(* Logix 5000 AddOnInstructionDefinition export EH_AL1323_8P_CommAOI; software revision 35.00 *)

TYPE EH_CommAOI_Data :
STRUCT
   Device_Comm_Error : BOOL;
   CommSuccess : BOOL;
   CommFailed : BOOL;
   CommTimeOut : BOOL;
   StateDone : BOOL;
   NewState : BOOL;
   OldState : SINT;
   PortSize : SINT;
   DevicePort : SINT;
   MaxState : SINT;
   State : SINT;
   VendorID : INT;
   DeviceID : DINT;
   CyclicData : INT[16];
   AcyclicData : DINT[8];
   ReplayIndex : INT;
   AOI_Diagnostic : DINT;
   ConnectionStatus : DINT;
   OutputData : INT[16];
END_STRUCT
END_TYPE

ADD_ON_INSTRUCTION EH_AL1323_8P_CommAOI   (* revision 1.0, vendor Endress+Hauser *)
// Ethenet/IP Comm AOI for 8 Port IFM AL 1323
// Revision note:
// First release of the IFM CommAOI with no array in the Tag Structure.
VAR_IN_OUT
   Master_InputTag : _0142:AL1323_43F9D57A:I:0; {required}
   Master_OutputTag : _0142:AL1323_F1871E46:O:0; {required}
   DataToSend : INT[10]; {required}
   CommAOIBusy : DINT; {required}
   ActiveComPort : DINT; {required}
   Send_Request : DINT; {required}
   CommError : INT; {required}
   DeviceData : EH_CommAOI_Data; {required}
END_VAR
VAR_INPUT
   iPortSize : INT; {required}
   iDevicePort : INT; {required}
   Master_Input_ConnectionFaulted : BOOL; {required}
END_VAR
VAR
   LocalChannel : DINT; {access None}
   LocalStep : DINT; {access None}
   cChannel : DINT; {access None}
   Port : SINT; {access None}
   count : SINT; {access None}
   PortSize : INT; {access None}
   ChannelData : DINT[15]; {access None}
   TONR_01 : FBD_TIMER; {access None}
   Calc_ConnectionStatus : INT; {access None}
   Calc_VID : INT; {access None}
   Calc_DID : INT; {access None}
   UsedState : INT; {access None}
   DataSendExecuted : BOOL; {access None}
   DataSize : SINT; {access None}
   RW_Input : SINT; {access None}
   RW_Step : SINT; {access None}
   TimerActive : BOOL; {access None}
   ExecuteCounter : DINT; {access None}
END_VAR

ROUTINE Logic   (* structured text *)
   //Create the Port Config 8P
   if iDevicePort > 0 and iDevicePort<9 then
   DeviceData.DevicePort := iDevicePort;
   else
   DeviceData.DevicePort := 0;
   end_if;
   
   DeviceData.PortSize := iPortSize;
   DeviceData.Device_Comm_Error := Master_Input_ConnectionFaulted;
   
   case DeviceData.PortSize of
   
   	0:
   		PortSize:= 1;
   	1:
   		PortSize:= 2;
   	2:
   		PortSize:= 4;
   	3:
   		PortSize:= 8;
   	4:
   		PortSize:= 16; //16 Int = 32Byte
   
   		DeviceData.AOI_Diagnostic.0 := 0;
   
   	else
   
   		DeviceData.AOI_Diagnostic.0 := 1;
   
   end_case;
   
   case DeviceData.DevicePort of
   
   	1:
   		//*********************************
   		//Device Connection Status within the Master
   		//*********************************
   
   		if Master_InputTag.Input_Data24 = 1
   		or Master_InputTag.Input_Data24 = 129 then
   
   			DeviceData.ConnectionStatus := 1; //Good
   
   		else
   
   			DeviceData.ConnectionStatus := 2; //Bad
   
   		end_if;
   
   		//*********************************
   		//Vendor ID
   		//*********************************
   
   		DeviceData.VendorID		:= Master_InputTag.Input_Data25;
   		DeviceData.VendorID.8	:= Master_InputTag.Input_Data25.8;
   		DeviceData.VendorID.9	:= Master_InputTag.Input_Data25.9;
   		DeviceData.VendorID.10	:= Master_InputTag.Input_Data25.10;
   		DeviceData.VendorID.11	:= Master_InputTag.Input_Data25.11;
   		DeviceData.VendorID.12	:= Master_InputTag.Input_Data25.12;
   		DeviceData.VendorID.13	:= Master_InputTag.Input_Data25.13;
   		DeviceData.VendorID.14	:= Master_InputTag.Input_Data25.14;
   		DeviceData.VendorID.15	:= Master_InputTag.Input_Data25.15;
   
   		//*********************************
   		//Device ID
   		//*********************************
   
   		DeviceData.DeviceID		:= Master_InputTag.Input_Data26;
   		DeviceData.DeviceID.8	:= Master_InputTag.Input_Data26.8;
   		DeviceData.DeviceID.9	:= Master_InputTag.Input_Data26.9;
   		DeviceData.DeviceID.10	:= Master_InputTag.Input_Data26.10;
   		DeviceData.DeviceID.11	:= Master_InputTag.Input_Data26.11;
   		DeviceData.DeviceID.12	:= Master_InputTag.Input_Data26.12;
   		DeviceData.DeviceID.13	:= Master_InputTag.Input_Data26.13;
   		DeviceData.DeviceID.14	:= Master_InputTag.Input_Data26.14;
   		DeviceData.DeviceID.15	:= Master_InputTag.Input_Data26.15;
   		DeviceData.DeviceID.16	:= Master_InputTag.Input_Data27.0;
   		DeviceData.DeviceID.17	:= Master_InputTag.Input_Data27.1;
   		DeviceData.DeviceID.18	:= Master_InputTag.Input_Data27.2;
   		DeviceData.DeviceID.19	:= Master_InputTag.Input_Data27.3;
   		DeviceData.DeviceID.20	:= Master_InputTag.Input_Data27.4;
   		DeviceData.DeviceID.21	:= Master_InputTag.Input_Data27.5;
   		DeviceData.DeviceID.22	:= Master_InputTag.Input_Data27.6;
   		DeviceData.DeviceID.23	:= Master_InputTag.Input_Data27.7;
   
   		//*********************************
   		//Cyclic Data Input
   		//*********************************
   
   		DeviceData.CyclicData[0] := Master_InputTag.Input_Data96;
   		DeviceData.CyclicData[1] := Master_InputTag.Input_Data97;
   		DeviceData.CyclicData[2] := Master_InputTag.Input_Data98;
   		DeviceData.CyclicData[3] := Master_InputTag.Input_Data99;
   		DeviceData.CyclicData[4] := Master_InputTag.Input_Data100;
   		DeviceData.CyclicData[5] := Master_InputTag.Input_Data101;
   		DeviceData.CyclicData[6] := Master_InputTag.Input_Data102;
   		DeviceData.CyclicData[7] := Master_InputTag.Input_Data103;
   		DeviceData.CyclicData[8] := Master_InputTag.Input_Data104;
   		DeviceData.CyclicData[9] := Master_InputTag.Input_Data105;
   		DeviceData.CyclicData[10] := Master_InputTag.Input_Data106;
   		DeviceData.CyclicData[11] := Master_InputTag.Input_Data107;
   		DeviceData.CyclicData[12] := Master_InputTag.Input_Data108;
   		DeviceData.CyclicData[13] := Master_InputTag.Input_Data109;
   		DeviceData.CyclicData[14] := Master_InputTag.Input_Data110;
   		DeviceData.CyclicData[15] := Master_InputTag.Input_Data111;
   
   
   		//*********************************
   		//Cyclic Data Output
   		//*********************************
   
   		Master_OutputTag.Output_Data24 := DeviceData.OutputData[0];
   		Master_OutputTag.Output_Data25 := DeviceData.OutputData[1];
   		Master_OutputTag.Output_Data26 := DeviceData.OutputData[2];
   		Master_OutputTag.Output_Data27 := DeviceData.OutputData[3];
   		Master_OutputTag.Output_Data28 := DeviceData.OutputData[4];
   		Master_OutputTag.Output_Data29 := DeviceData.OutputData[5];
   		Master_OutputTag.Output_Data30 := DeviceData.OutputData[6];
   		Master_OutputTag.Output_Data31 := DeviceData.OutputData[7];
   		Master_OutputTag.Output_Data32 := DeviceData.OutputData[8];
   		Master_OutputTag.Output_Data33 := DeviceData.OutputData[9];
   		Master_OutputTag.Output_Data34 := DeviceData.OutputData[10];
   		Master_OutputTag.Output_Data35 := DeviceData.OutputData[11];
   		Master_OutputTag.Output_Data36 := DeviceData.OutputData[12];
   		Master_OutputTag.Output_Data37 := DeviceData.OutputData[13];
   		Master_OutputTag.Output_Data38 := DeviceData.OutputData[14];
   		Master_OutputTag.Output_Data39 := DeviceData.OutputData[15];
   
   	2:
   		//*********************************
   		//Device Connection Status within the Master
   		//*********************************
   
   		if Master_InputTag.Input_Data33 = 1
   		or Master_InputTag.Input_Data33 = 129 then
   
   			DeviceData.ConnectionStatus := 1; //Good
   
   		else
   
   			DeviceData.ConnectionStatus := 2; //Bad
   
   		end_if;
   
   		//*********************************
   		//Vendor ID
   		//*********************************
   
   		DeviceData.VendorID		:= Master_InputTag.Input_Data34;
   		DeviceData.VendorID.8	:= Master_InputTag.Input_Data34.8;
   		DeviceData.VendorID.9	:= Master_InputTag.Input_Data34.9;
   		DeviceData.VendorID.10	:= Master_InputTag.Input_Data34.10;
   		DeviceData.VendorID.11	:= Master_InputTag.Input_Data34.11;
   		DeviceData.VendorID.12	:= Master_InputTag.Input_Data34.12;
   		DeviceData.VendorID.13	:= Master_InputTag.Input_Data34.13;
   		DeviceData.VendorID.14	:= Master_InputTag.Input_Data34.14;
   		DeviceData.VendorID.15	:= Master_InputTag.Input_Data34.15;
   
   		//*********************************
   		//Device ID
   		//*********************************
   
   		DeviceData.DeviceID		:= Master_InputTag.Input_Data35;
   		DeviceData.DeviceID.8	:= Master_InputTag.Input_Data35.8;
   		DeviceData.DeviceID.9	:= Master_InputTag.Input_Data35.9;
   		DeviceData.DeviceID.10	:= Master_InputTag.Input_Data35.10;
   		DeviceData.DeviceID.11	:= Master_InputTag.Input_Data35.11;
   		DeviceData.DeviceID.12	:= Master_InputTag.Input_Data35.12;
   		DeviceData.DeviceID.13	:= Master_InputTag.Input_Data35.13;
   		DeviceData.DeviceID.14	:= Master_InputTag.Input_Data35.14;
   		DeviceData.DeviceID.15	:= Master_InputTag.Input_Data35.15;
   		DeviceData.DeviceID.16	:= Master_InputTag.Input_Data36.0;
   		DeviceData.DeviceID.17	:= Master_InputTag.Input_Data36.1;
   		DeviceData.DeviceID.18	:= Master_InputTag.Input_Data36.2;
   		DeviceData.DeviceID.19	:= Master_InputTag.Input_Data36.3;
   		DeviceData.DeviceID.20	:= Master_InputTag.Input_Data36.4;
   		DeviceData.DeviceID.21	:= Master_InputTag.Input_Data36.5;
   		DeviceData.DeviceID.22	:= Master_InputTag.Input_Data36.6;
   		DeviceData.DeviceID.23	:= Master_InputTag.Input_Data36.7;
   
   		//*********************************
   		//Cyclic Data Input
   		//*********************************
   
   		DeviceData.CyclicData[0] := Master_InputTag.Input_Data112;
   		DeviceData.CyclicData[1] := Master_InputTag.Input_Data113;
   		DeviceData.CyclicData[2] := Master_InputTag.Input_Data114;
   		DeviceData.CyclicData[3] := Master_InputTag.Input_Data115;
   		DeviceData.CyclicData[4] := Master_InputTag.Input_Data116;
   		DeviceData.CyclicData[5] := Master_InputTag.Input_Data117;
   		DeviceData.CyclicData[6] := Master_InputTag.Input_Data118;
   		DeviceData.CyclicData[7] := Master_InputTag.Input_Data119;
   		DeviceData.CyclicData[8] := Master_InputTag.Input_Data120;
   		DeviceData.CyclicData[9] := Master_InputTag.Input_Data121;
   		DeviceData.CyclicData[10] := Master_InputTag.Input_Data122;
   		DeviceData.CyclicData[11] := Master_InputTag.Input_Data123;
   		DeviceData.CyclicData[12] := Master_InputTag.Input_Data124;
   		DeviceData.CyclicData[13] := Master_InputTag.Input_Data125;
   		DeviceData.CyclicData[14] := Master_InputTag.Input_Data126;
   		DeviceData.CyclicData[15] := Master_InputTag.Input_Data127;
   
   		//*********************************
   		//Cyclic Data Output
   		//*********************************
   
   		Master_OutputTag.Output_Data40 := DeviceData.OutputData[0];
   		Master_OutputTag.Output_Data41 := DeviceData.OutputData[1];
   		Master_OutputTag.Output_Data42 := DeviceData.OutputData[2];
   		Master_OutputTag.Output_Data43 := DeviceData.OutputData[3];
   		Master_OutputTag.Output_Data44 := DeviceData.OutputData[4];
   		Master_OutputTag.Output_Data45 := DeviceData.OutputData[5];
   		Master_OutputTag.Output_Data46 := DeviceData.OutputData[6];
   		Master_OutputTag.Output_Data47 := DeviceData.OutputData[7];
   		Master_OutputTag.Output_Data48 := DeviceData.OutputData[8];
   		Master_OutputTag.Output_Data49 := DeviceData.OutputData[9];
   		Master_OutputTag.Output_Data50 := DeviceData.OutputData[10];
   		Master_OutputTag.Output_Data51 := DeviceData.OutputData[11];
   		Master_OutputTag.Output_Data52 := DeviceData.OutputData[12];
   		Master_OutputTag.Output_Data53 := DeviceData.OutputData[13];
   		Master_OutputTag.Output_Data54 := DeviceData.OutputData[14];
   		Master_OutputTag.Output_Data55 := DeviceData.OutputData[15];
   
   	3:
   		//*********************************
   		//Device Connection Status within the Master
   		//*********************************
   
   		if Master_InputTag.Input_Data42 = 1
   		or Master_InputTag.Input_Data42 = 129 then
   
   			DeviceData.ConnectionStatus := 1; //Good
   
   		else
   
   			DeviceData.ConnectionStatus := 2; //Bad
   
   		end_if;
   
   		//*********************************
   		//Vendor ID
   		//*********************************
   
   		DeviceData.VendorID		:= Master_InputTag.Input_Data43;
   		DeviceData.VendorID.8	:= Master_InputTag.Input_Data43.8;
   		DeviceData.VendorID.9	:= Master_InputTag.Input_Data43.9;
   		DeviceData.VendorID.10	:= Master_InputTag.Input_Data43.10;
   		DeviceData.VendorID.11	:= Master_InputTag.Input_Data43.11;
   		DeviceData.VendorID.12	:= Master_InputTag.Input_Data43.12;
   		DeviceData.VendorID.13	:= Master_InputTag.Input_Data43.13;
   		DeviceData.VendorID.14	:= Master_InputTag.Input_Data43.14;
   		DeviceData.VendorID.15	:= Master_InputTag.Input_Data43.15;
   
   		//*********************************
   		//Device ID
   		//*********************************
   
   		DeviceData.DeviceID		:= Master_InputTag.Input_Data44;
   		DeviceData.DeviceID.8	:= Master_InputTag.Input_Data44.8;
   		DeviceData.DeviceID.9	:= Master_InputTag.Input_Data44.9;
   		DeviceData.DeviceID.10	:= Master_InputTag.Input_Data44.10;
   		DeviceData.DeviceID.11	:= Master_InputTag.Input_Data44.11;
   		DeviceData.DeviceID.12	:= Master_InputTag.Input_Data44.12;
   		DeviceData.DeviceID.13	:= Master_InputTag.Input_Data44.13;
   		DeviceData.DeviceID.14	:= Master_InputTag.Input_Data44.14;
   		DeviceData.DeviceID.15	:= Master_InputTag.Input_Data44.15;
   		DeviceData.DeviceID.16	:= Master_InputTag.Input_Data45.0;
   		DeviceData.DeviceID.17	:= Master_InputTag.Input_Data45.1;
   		DeviceData.DeviceID.18	:= Master_InputTag.Input_Data45.2;
   		DeviceData.DeviceID.19	:= Master_InputTag.Input_Data45.3;
   		DeviceData.DeviceID.20	:= Master_InputTag.Input_Data45.4;
   		DeviceData.DeviceID.21	:= Master_InputTag.Input_Data45.5;
   		DeviceData.DeviceID.22	:= Master_InputTag.Input_Data45.6;
   		DeviceData.DeviceID.23	:= Master_InputTag.Input_Data45.7;
   
   		//*********************************
   		//Cyclic Data Input
   		//*********************************
   
   		DeviceData.CyclicData[0] := Master_InputTag.Input_Data128;
   		DeviceData.CyclicData[1] := Master_InputTag.Input_Data129;
   		DeviceData.CyclicData[2] := Master_InputTag.Input_Data130;
   		DeviceData.CyclicData[3] := Master_InputTag.Input_Data131;
   		DeviceData.CyclicData[4] := Master_InputTag.Input_Data132;
   		DeviceData.CyclicData[5] := Master_InputTag.Input_Data133;
   		DeviceData.CyclicData[6] := Master_InputTag.Input_Data134;
   		DeviceData.CyclicData[7] := Master_InputTag.Input_Data135;
   		DeviceData.CyclicData[8] := Master_InputTag.Input_Data136;
   		DeviceData.CyclicData[9] := Master_InputTag.Input_Data137;
   		DeviceData.CyclicData[10] := Master_InputTag.Input_Data138;
   		DeviceData.CyclicData[11] := Master_InputTag.Input_Data139;
   		DeviceData.CyclicData[12] := Master_InputTag.Input_Data140;
   		DeviceData.CyclicData[13] := Master_InputTag.Input_Data141;
   		DeviceData.CyclicData[14] := Master_InputTag.Input_Data142;
   		DeviceData.CyclicData[15] := Master_InputTag.Input_Data143;
   
   		//*********************************
   		//Cyclic Data Output
   		//*********************************
   
   		Master_OutputTag.Output_Data56 := DeviceData.OutputData[0];
   		Master_OutputTag.Output_Data58 := DeviceData.OutputData[2];
   		Master_OutputTag.Output_Data59 := DeviceData.OutputData[3];
   		Master_OutputTag.Output_Data60 := DeviceData.OutputData[4];
   		Master_OutputTag.Output_Data61 := DeviceData.OutputData[5];
   		Master_OutputTag.Output_Data57 := DeviceData.OutputData[1];
   		Master_OutputTag.Output_Data62 := DeviceData.OutputData[6];
   		Master_OutputTag.Output_Data63 := DeviceData.OutputData[7];
   		Master_OutputTag.Output_Data64 := DeviceData.OutputData[8];
   		Master_OutputTag.Output_Data65 := DeviceData.OutputData[9];
   		Master_OutputTag.Output_Data66 := DeviceData.OutputData[10];
   		Master_OutputTag.Output_Data67 := DeviceData.OutputData[11];
   		Master_OutputTag.Output_Data68 := DeviceData.OutputData[12];
   		Master_OutputTag.Output_Data69 := DeviceData.OutputData[13];
   		Master_OutputTag.Output_Data70 := DeviceData.OutputData[14];
   		Master_OutputTag.Output_Data71 := DeviceData.OutputData[15];
   
   	4:
   		//*********************************
   		//Device Connection Status within the Master
   		//*********************************
   
   		if Master_InputTag.Input_Data51 = 1
   		or Master_InputTag.Input_Data51 = 129 then
   
   			DeviceData.ConnectionStatus := 1; //Good
   
   		else
   
   			DeviceData.ConnectionStatus := 2; //Bad
   
   		end_if;
   
   		//*********************************
   		//Vendor ID
   		//*********************************
   
   		DeviceData.VendorID		:= Master_InputTag.Input_Data52;
   		DeviceData.VendorID.8	:= Master_InputTag.Input_Data52.8;
   		DeviceData.VendorID.9	:= Master_InputTag.Input_Data52.9;
   		DeviceData.VendorID.10	:= Master_InputTag.Input_Data52.10;
   		DeviceData.VendorID.11	:= Master_InputTag.Input_Data52.11;
   		DeviceData.VendorID.12	:= Master_InputTag.Input_Data52.12;
   		DeviceData.VendorID.13	:= Master_InputTag.Input_Data52.13;
   		DeviceData.VendorID.14	:= Master_InputTag.Input_Data52.14;
   		DeviceData.VendorID.15	:= Master_InputTag.Input_Data52.15;
   
   		//*********************************
   		//Device ID
   		//*********************************
   
   		DeviceData.DeviceID		:= Master_InputTag.Input_Data53;
   		DeviceData.DeviceID.8	:= Master_InputTag.Input_Data53.8;
   		DeviceData.DeviceID.9	:= Master_InputTag.Input_Data53.9;
   		DeviceData.DeviceID.10	:= Master_InputTag.Input_Data53.10;
   		DeviceData.DeviceID.11	:= Master_InputTag.Input_Data53.11;
   		DeviceData.DeviceID.12	:= Master_InputTag.Input_Data53.12;
   		DeviceData.DeviceID.13	:= Master_InputTag.Input_Data53.13;
   		DeviceData.DeviceID.14	:= Master_InputTag.Input_Data53.14;
   		DeviceData.DeviceID.15	:= Master_InputTag.Input_Data53.15;
   		DeviceData.DeviceID.16	:= Master_InputTag.Input_Data54.0;
   		DeviceData.DeviceID.17	:= Master_InputTag.Input_Data54.1;
   		DeviceData.DeviceID.18	:= Master_InputTag.Input_Data54.2;
   		DeviceData.DeviceID.19	:= Master_InputTag.Input_Data54.3;
   		DeviceData.DeviceID.20	:= Master_InputTag.Input_Data54.4;
   		DeviceData.DeviceID.21	:= Master_InputTag.Input_Data54.5;
   		DeviceData.DeviceID.22	:= Master_InputTag.Input_Data54.6;
   		DeviceData.DeviceID.23	:= Master_InputTag.Input_Data54.7;
   
   		//*********************************
   		//Cyclic Data Input
   		//*********************************
   
   		DeviceData.CyclicData[0] := Master_InputTag.Input_Data144;
   		DeviceData.CyclicData[1] := Master_InputTag.Input_Data145;
   		DeviceData.CyclicData[2] := Master_InputTag.Input_Data146;
   		DeviceData.CyclicData[3] := Master_InputTag.Input_Data147;
   		DeviceData.CyclicData[4] := Master_InputTag.Input_Data148;
   		DeviceData.CyclicData[5] := Master_InputTag.Input_Data149;
   		DeviceData.CyclicData[6] := Master_InputTag.Input_Data150;
   		DeviceData.CyclicData[7] := Master_InputTag.Input_Data151;
   		DeviceData.CyclicData[8] := Master_InputTag.Input_Data152;
   		DeviceData.CyclicData[9] := Master_InputTag.Input_Data153;
   		DeviceData.CyclicData[10] := Master_InputTag.Input_Data154;
   		DeviceData.CyclicData[11] := Master_InputTag.Input_Data155;
   		DeviceData.CyclicData[12] := Master_InputTag.Input_Data156;
   		DeviceData.CyclicData[13] := Master_InputTag.Input_Data157;
   		DeviceData.CyclicData[14] := Master_InputTag.Input_Data158;
   		DeviceData.CyclicData[15] := Master_InputTag.Input_Data159;
   
   		//*********************************
   		//Cyclic Data Output
   		//*********************************
   
   		Master_OutputTag.Output_Data72 := DeviceData.OutputData[0];
   		Master_OutputTag.Output_Data73 := DeviceData.OutputData[1];
   		Master_OutputTag.Output_Data74 := DeviceData.OutputData[2];
   		Master_OutputTag.Output_Data75 := DeviceData.OutputData[3];
   		Master_OutputTag.Output_Data76 := DeviceData.OutputData[4];
   		Master_OutputTag.Output_Data77 := DeviceData.OutputData[5];
   		Master_OutputTag.Output_Data78 := DeviceData.OutputData[6];
   		Master_OutputTag.Output_Data79 := DeviceData.OutputData[7];
   		Master_OutputTag.Output_Data80 := DeviceData.OutputData[8];
   		Master_OutputTag.Output_Data81 := DeviceData.OutputData[9];
   		Master_OutputTag.Output_Data82 := DeviceData.OutputData[10];
   		Master_OutputTag.Output_Data83 := DeviceData.OutputData[11];
   		Master_OutputTag.Output_Data84 := DeviceData.OutputData[12];
   		Master_OutputTag.Output_Data85 := DeviceData.OutputData[13];
   		Master_OutputTag.Output_Data86 := DeviceData.OutputData[14];
   		Master_OutputTag.Output_Data87 := DeviceData.OutputData[15];
   
   	5:
   		//*********************************
   		//Device Connection Status within the Master
   		//*********************************
   
   		if Master_InputTag.Input_Data60 = 1
   		or Master_InputTag.Input_Data60 = 129 then
   
   			DeviceData.ConnectionStatus := 1; //Good
   
   		else
   
   			DeviceData.ConnectionStatus := 2; //Bad
   
   		end_if;
   
   		//*********************************
   		//Vendor ID
   		//*********************************
   
   		DeviceData.VendorID		:= Master_InputTag.Input_Data61;
   		DeviceData.VendorID.8	:= Master_InputTag.Input_Data61.8;
   		DeviceData.VendorID.9	:= Master_InputTag.Input_Data61.9;
   		DeviceData.VendorID.10	:= Master_InputTag.Input_Data61.10;
   		DeviceData.VendorID.11	:= Master_InputTag.Input_Data61.11;
   		DeviceData.VendorID.12	:= Master_InputTag.Input_Data61.12;
   		DeviceData.VendorID.13	:= Master_InputTag.Input_Data61.13;
   		DeviceData.VendorID.14	:= Master_InputTag.Input_Data61.14;
   		DeviceData.VendorID.15	:= Master_InputTag.Input_Data61.15;
   
   		//*********************************
   		//Device ID
   		//*********************************
   
   		DeviceData.DeviceID		:= Master_InputTag.Input_Data62;
   		DeviceData.DeviceID.8	:= Master_InputTag.Input_Data62.8;
   		DeviceData.DeviceID.9	:= Master_InputTag.Input_Data62.9;
   		DeviceData.DeviceID.10	:= Master_InputTag.Input_Data62.10;
   		DeviceData.DeviceID.11	:= Master_InputTag.Input_Data62.11;
   		DeviceData.DeviceID.12	:= Master_InputTag.Input_Data62.12;
   		DeviceData.DeviceID.13	:= Master_InputTag.Input_Data62.13;
   		DeviceData.DeviceID.14	:= Master_InputTag.Input_Data62.14;
   		DeviceData.DeviceID.15	:= Master_InputTag.Input_Data62.15;
   		DeviceData.DeviceID.16	:= Master_InputTag.Input_Data63.0;
   		DeviceData.DeviceID.17	:= Master_InputTag.Input_Data63.1;
   		DeviceData.DeviceID.18	:= Master_InputTag.Input_Data63.2;
   		DeviceData.DeviceID.19	:= Master_InputTag.Input_Data63.3;
   		DeviceData.DeviceID.20	:= Master_InputTag.Input_Data63.4;
   		DeviceData.DeviceID.21	:= Master_InputTag.Input_Data63.5;
   		DeviceData.DeviceID.22	:= Master_InputTag.Input_Data63.6;
   		DeviceData.DeviceID.23	:= Master_InputTag.Input_Data63.7;
   
   		//*********************************
   		//Cyclic Data Input
   		//*********************************
   
   		DeviceData.CyclicData[0] := Master_InputTag.Input_Data160;
   		DeviceData.CyclicData[1] := Master_InputTag.Input_Data161;
   		DeviceData.CyclicData[2] := Master_InputTag.Input_Data162;
   		DeviceData.CyclicData[3] := Master_InputTag.Input_Data163;
   		DeviceData.CyclicData[4] := Master_InputTag.Input_Data164;
   		DeviceData.CyclicData[5] := Master_InputTag.Input_Data165;
   		DeviceData.CyclicData[6] := Master_InputTag.Input_Data166;
   		DeviceData.CyclicData[7] := Master_InputTag.Input_Data167;
   		DeviceData.CyclicData[8] := Master_InputTag.Input_Data168;
   		DeviceData.CyclicData[9] := Master_InputTag.Input_Data169;
   		DeviceData.CyclicData[10] := Master_InputTag.Input_Data170;
   		DeviceData.CyclicData[11] := Master_InputTag.Input_Data171;
   		DeviceData.CyclicData[12] := Master_InputTag.Input_Data172;
   		DeviceData.CyclicData[13] := Master_InputTag.Input_Data173;
   		DeviceData.CyclicData[14] := Master_InputTag.Input_Data174;
   		DeviceData.CyclicData[15] := Master_InputTag.Input_Data175;
   
   		//*********************************
   		//Cyclic Data Output
   		//*********************************
   
   		Master_OutputTag.Output_Data88 := DeviceData.OutputData[0];
   		Master_OutputTag.Output_Data89 := DeviceData.OutputData[1];
   		Master_OutputTag.Output_Data90 := DeviceData.OutputData[2];
   		Master_OutputTag.Output_Data91 := DeviceData.OutputData[3];
   		Master_OutputTag.Output_Data92 := DeviceData.OutputData[4];
   		Master_OutputTag.Output_Data93 := DeviceData.OutputData[5];
   		Master_OutputTag.Output_Data94 := DeviceData.OutputData[6];
   		Master_OutputTag.Output_Data95 := DeviceData.OutputData[7];
   		Master_OutputTag.Output_Data96 := DeviceData.OutputData[8];
   		Master_OutputTag.Output_Data97 := DeviceData.OutputData[9];
   		Master_OutputTag.Output_Data98 := DeviceData.OutputData[10];
   		Master_OutputTag.Output_Data99 := DeviceData.OutputData[11];
   		Master_OutputTag.Output_Data100 := DeviceData.OutputData[12];
   		Master_OutputTag.Output_Data101 := DeviceData.OutputData[13];
   		Master_OutputTag.Output_Data102 := DeviceData.OutputData[14];
   		Master_OutputTag.Output_Data103 := DeviceData.OutputData[15];
   
   	6:
   		//*******************************************
   		//Device Connection Status within the Master
   		//*******************************************
   
   		if Master_InputTag.Input_Data69 = 1
   		or Master_InputTag.Input_Data69 = 129 then
   
   			DeviceData.ConnectionStatus := 1; //Good
   
   		else
   
   			DeviceData.ConnectionStatus := 2; //Bad
   
   		end_if;
   
   		//*********************************
   		//Vendor ID
   		//*********************************
   
   		DeviceData.VendorID		:= Master_InputTag.Input_Data70;
   		DeviceData.VendorID.8	:= Master_InputTag.Input_Data70.8;
   		DeviceData.VendorID.9	:= Master_InputTag.Input_Data70.9;
   		DeviceData.VendorID.10	:= Master_InputTag.Input_Data70.10;
   		DeviceData.VendorID.11	:= Master_InputTag.Input_Data70.11;
   		DeviceData.VendorID.12	:= Master_InputTag.Input_Data70.12;
   		DeviceData.VendorID.13	:= Master_InputTag.Input_Data70.13;
   		DeviceData.VendorID.14	:= Master_InputTag.Input_Data70.14;
   		DeviceData.VendorID.15	:= Master_InputTag.Input_Data70.15;
   
   		//*********************************
   		//Device ID
   		//*********************************
   
   		DeviceData.DeviceID		:= Master_InputTag.Input_Data71;
   		DeviceData.DeviceID.8	:= Master_InputTag.Input_Data71.8;
   		DeviceData.DeviceID.9	:= Master_InputTag.Input_Data71.9;
   		DeviceData.DeviceID.10	:= Master_InputTag.Input_Data71.10;
   		DeviceData.DeviceID.11	:= Master_InputTag.Input_Data71.11;
   		DeviceData.DeviceID.12	:= Master_InputTag.Input_Data71.12;
   		DeviceData.DeviceID.13	:= Master_InputTag.Input_Data71.13;
   		DeviceData.DeviceID.14	:= Master_InputTag.Input_Data71.14;
   		DeviceData.DeviceID.15	:= Master_InputTag.Input_Data71.15;
   		DeviceData.DeviceID.16	:= Master_InputTag.Input_Data72.0;
   		DeviceData.DeviceID.17	:= Master_InputTag.Input_Data72.1;
   		DeviceData.DeviceID.18	:= Master_InputTag.Input_Data72.2;
   		DeviceData.DeviceID.19	:= Master_InputTag.Input_Data72.3;
   		DeviceData.DeviceID.20	:= Master_InputTag.Input_Data72.4;
   		DeviceData.DeviceID.21	:= Master_InputTag.Input_Data72.5;
   		DeviceData.DeviceID.22	:= Master_InputTag.Input_Data72.6;
   		DeviceData.DeviceID.23	:= Master_InputTag.Input_Data72.7;
   
   		//*********************************
   		//Cyclic Data Input
   		//*********************************
   
   		DeviceData.CyclicData[0] := Master_InputTag.Input_Data176;
   		DeviceData.CyclicData[1] := Master_InputTag.Input_Data177;
   		DeviceData.CyclicData[2] := Master_InputTag.Input_Data178;
   		DeviceData.CyclicData[3] := Master_InputTag.Input_Data179;
   		DeviceData.CyclicData[4] := Master_InputTag.Input_Data180;
   		DeviceData.CyclicData[5] := Master_InputTag.Input_Data181;
   		DeviceData.CyclicData[6] := Master_InputTag.Input_Data182;
   		DeviceData.CyclicData[7] := Master_InputTag.Input_Data183;
   		DeviceData.CyclicData[8] := Master_InputTag.Input_Data184;
   		DeviceData.CyclicData[9] := Master_InputTag.Input_Data185;
   		DeviceData.CyclicData[10] := Master_InputTag.Input_Data186;
   		DeviceData.CyclicData[11] := Master_InputTag.Input_Data187;
   		DeviceData.CyclicData[12] := Master_InputTag.Input_Data188;
   		DeviceData.CyclicData[13] := Master_InputTag.Input_Data189;
   		DeviceData.CyclicData[14] := Master_InputTag.Input_Data190;
   		DeviceData.CyclicData[15] := Master_InputTag.Input_Data191;
   
   		//*********************************
   		//Cyclic Data Output
   		//*********************************
   
   		Master_OutputTag.Output_Data104 := DeviceData.OutputData[0];
   		Master_OutputTag.Output_Data105 := DeviceData.OutputData[1];
   		Master_OutputTag.Output_Data106 := DeviceData.OutputData[2];
   		Master_OutputTag.Output_Data107 := DeviceData.OutputData[3];
   		Master_OutputTag.Output_Data108 := DeviceData.OutputData[4];
   		Master_OutputTag.Output_Data109 := DeviceData.OutputData[5];
   		Master_OutputTag.Output_Data110 := DeviceData.OutputData[6];
   		Master_OutputTag.Output_Data111 := DeviceData.OutputData[7];
   		Master_OutputTag.Output_Data112 := DeviceData.OutputData[8];
   		Master_OutputTag.Output_Data113 := DeviceData.OutputData[9];
   		Master_OutputTag.Output_Data114 := DeviceData.OutputData[10];
   		Master_OutputTag.Output_Data115 := DeviceData.OutputData[11];
   		Master_OutputTag.Output_Data116 := DeviceData.OutputData[12];
   		Master_OutputTag.Output_Data117 := DeviceData.OutputData[13];
   		Master_OutputTag.Output_Data118 := DeviceData.OutputData[14];
   		Master_OutputTag.Output_Data119 := DeviceData.OutputData[15];
   
   	7:
   		//*******************************************
   		//Device Connection Status within the Master
   		//*******************************************
   
   		if Master_InputTag.Input_Data78 = 1
   		or Master_InputTag.Input_Data78 = 129 then
   
   			DeviceData.ConnectionStatus := 1; //Good
   
   		else
   
   			DeviceData.ConnectionStatus := 2; //Bad
   
   		end_if;
   
   		//*********************************
   		//Vendor ID
   		//*********************************
   
   		DeviceData.VendorID		:= Master_InputTag.Input_Data79;
   		DeviceData.VendorID.8	:= Master_InputTag.Input_Data79.8;
   		DeviceData.VendorID.9	:= Master_InputTag.Input_Data79.9;
   		DeviceData.VendorID.10	:= Master_InputTag.Input_Data79.10;
   		DeviceData.VendorID.11	:= Master_InputTag.Input_Data79.11;
   		DeviceData.VendorID.12	:= Master_InputTag.Input_Data79.12;
   		DeviceData.VendorID.13	:= Master_InputTag.Input_Data79.13;
   		DeviceData.VendorID.14	:= Master_InputTag.Input_Data79.14;
   		DeviceData.VendorID.15	:= Master_InputTag.Input_Data79.15;
   
   		//*********************************
   		//Device ID
   		//*********************************
   
   		DeviceData.DeviceID		:= Master_InputTag.Input_Data80;
   		DeviceData.DeviceID.8	:= Master_InputTag.Input_Data80.8;
   		DeviceData.DeviceID.9	:= Master_InputTag.Input_Data80.9;
   		DeviceData.DeviceID.10	:= Master_InputTag.Input_Data80.10;
   		DeviceData.DeviceID.11	:= Master_InputTag.Input_Data80.11;
   		DeviceData.DeviceID.12	:= Master_InputTag.Input_Data80.12;
   		DeviceData.DeviceID.13	:= Master_InputTag.Input_Data80.13;
   		DeviceData.DeviceID.14	:= Master_InputTag.Input_Data80.14;
   		DeviceData.DeviceID.15	:= Master_InputTag.Input_Data80.15;
   		DeviceData.DeviceID.16	:= Master_InputTag.Input_Data81.0;
   		DeviceData.DeviceID.17	:= Master_InputTag.Input_Data81.1;
   		DeviceData.DeviceID.18	:= Master_InputTag.Input_Data81.2;
   		DeviceData.DeviceID.19	:= Master_InputTag.Input_Data81.3;
   		DeviceData.DeviceID.20	:= Master_InputTag.Input_Data81.4;
   		DeviceData.DeviceID.21	:= Master_InputTag.Input_Data81.5;
   		DeviceData.DeviceID.22	:= Master_InputTag.Input_Data81.6;
   		DeviceData.DeviceID.23	:= Master_InputTag.Input_Data81.7;
   
   		//*********************************
   		//Cyclic Data Input
   		//*********************************
   
   		DeviceData.CyclicData[0] := Master_InputTag.Input_Data192;
   		DeviceData.CyclicData[1] := Master_InputTag.Input_Data193;
   		DeviceData.CyclicData[2] := Master_InputTag.Input_Data194;
   		DeviceData.CyclicData[3] := Master_InputTag.Input_Data195;
   		DeviceData.CyclicData[4] := Master_InputTag.Input_Data196;
   		DeviceData.CyclicData[5] := Master_InputTag.Input_Data197;
   		DeviceData.CyclicData[6] := Master_InputTag.Input_Data198;
   		DeviceData.CyclicData[7] := Master_InputTag.Input_Data199;
   		DeviceData.CyclicData[8] := Master_InputTag.Input_Data200;
   		DeviceData.CyclicData[9] := Master_InputTag.Input_Data201;
   		DeviceData.CyclicData[10] := Master_InputTag.Input_Data202;
   		DeviceData.CyclicData[11] := Master_InputTag.Input_Data203;
   		DeviceData.CyclicData[12] := Master_InputTag.Input_Data204;
   		DeviceData.CyclicData[13] := Master_InputTag.Input_Data205;
   		DeviceData.CyclicData[14] := Master_InputTag.Input_Data206;
   		DeviceData.CyclicData[15] := Master_InputTag.Input_Data207;
   
   		//*********************************
   		//Cyclic Data Output
   		//*********************************
   
   		Master_OutputTag.Output_Data120 := DeviceData.OutputData[0];
   		Master_OutputTag.Output_Data121 := DeviceData.OutputData[1];
   		Master_OutputTag.Output_Data122 := DeviceData.OutputData[2];
   		Master_OutputTag.Output_Data123 := DeviceData.OutputData[3];
   		Master_OutputTag.Output_Data124 := DeviceData.OutputData[4];
   		Master_OutputTag.Output_Data125 := DeviceData.OutputData[5];
   		Master_OutputTag.Output_Data126 := DeviceData.OutputData[6];
   		Master_OutputTag.Output_Data127 := DeviceData.OutputData[7];
   		Master_OutputTag.Output_Data128 := DeviceData.OutputData[8];
   		Master_OutputTag.Output_Data129 := DeviceData.OutputData[9];
   		Master_OutputTag.Output_Data130 := DeviceData.OutputData[10];
   		Master_OutputTag.Output_Data131 := DeviceData.OutputData[11];
   		Master_OutputTag.Output_Data132 := DeviceData.OutputData[12];
   		Master_OutputTag.Output_Data133 := DeviceData.OutputData[13];
   		Master_OutputTag.Output_Data134 := DeviceData.OutputData[14];
   		Master_OutputTag.Output_Data135 := DeviceData.OutputData[15];
   
   	8:
   		//*********************************
   		//Device Connection Status within the Master
   		//*********************************
   
   		if Master_InputTag.Input_Data87 = 1
   		or Master_InputTag.Input_Data87 = 129 then
   
   			DeviceData.ConnectionStatus := 1; //Good
   
   		else
   
   			DeviceData.ConnectionStatus := 2; //Bad
   
   		end_if;
   
   		//*********************************
   		//Vendor ID
   		//*********************************
   
   		DeviceData.VendorID		:= Master_InputTag.Input_Data88;
   		DeviceData.VendorID.8	:= Master_InputTag.Input_Data88.8;
   		DeviceData.VendorID.9	:= Master_InputTag.Input_Data88.9;
   		DeviceData.VendorID.10	:= Master_InputTag.Input_Data88.10;
   		DeviceData.VendorID.11	:= Master_InputTag.Input_Data88.11;
   		DeviceData.VendorID.12	:= Master_InputTag.Input_Data88.12;
   		DeviceData.VendorID.13	:= Master_InputTag.Input_Data88.13;
   		DeviceData.VendorID.14	:= Master_InputTag.Input_Data88.14;
   		DeviceData.VendorID.15	:= Master_InputTag.Input_Data88.15;
   
   		//*********************************
   		//Device ID
   		//*********************************
   
   		DeviceData.DeviceID		:= Master_InputTag.Input_Data89;
   		DeviceData.DeviceID.8	:= Master_InputTag.Input_Data89.8;
   		DeviceData.DeviceID.9	:= Master_InputTag.Input_Data89.9;
   		DeviceData.DeviceID.10	:= Master_InputTag.Input_Data89.10;
   		DeviceData.DeviceID.11	:= Master_InputTag.Input_Data89.11;
   		DeviceData.DeviceID.12	:= Master_InputTag.Input_Data89.12;
   		DeviceData.DeviceID.13	:= Master_InputTag.Input_Data89.13;
   		DeviceData.DeviceID.14	:= Master_InputTag.Input_Data89.14;
   		DeviceData.DeviceID.15	:= Master_InputTag.Input_Data89.15;
   		DeviceData.DeviceID.16	:= Master_InputTag.Input_Data90.0;
   		DeviceData.DeviceID.17	:= Master_InputTag.Input_Data90.1;
   		DeviceData.DeviceID.18	:= Master_InputTag.Input_Data90.2;
   		DeviceData.DeviceID.19	:= Master_InputTag.Input_Data90.3;
   		DeviceData.DeviceID.20	:= Master_InputTag.Input_Data90.4;
   		DeviceData.DeviceID.21	:= Master_InputTag.Input_Data90.5;
   		DeviceData.DeviceID.22	:= Master_InputTag.Input_Data90.6;
   		DeviceData.DeviceID.23	:= Master_InputTag.Input_Data90.7;
   
   		//*********************************
   		//Cyclic Data Input
   		//*********************************
   
   		DeviceData.CyclicData[0] := Master_InputTag.Input_Data208;
   		DeviceData.CyclicData[1] := Master_InputTag.Input_Data209;
   		DeviceData.CyclicData[2] := Master_InputTag.Input_Data210;
   		DeviceData.CyclicData[3] := Master_InputTag.Input_Data211;
   		DeviceData.CyclicData[4] := Master_InputTag.Input_Data212;
   		DeviceData.CyclicData[5] := Master_InputTag.Input_Data213;
   		DeviceData.CyclicData[6] := Master_InputTag.Input_Data214;
   		DeviceData.CyclicData[7] := Master_InputTag.Input_Data215;
   		DeviceData.CyclicData[8] := Master_InputTag.Input_Data216;
   		DeviceData.CyclicData[9] := Master_InputTag.Input_Data217;
   		DeviceData.CyclicData[10] := Master_InputTag.Input_Data218;
   		DeviceData.CyclicData[11] := Master_InputTag.Input_Data219;
   		DeviceData.CyclicData[12] := Master_InputTag.Input_Data220;
   		DeviceData.CyclicData[13] := Master_InputTag.Input_Data221;
   		DeviceData.CyclicData[14] := Master_InputTag.Input_Data222;
   		DeviceData.CyclicData[15] := Master_InputTag.Input_Data223;
   
   
   		//*********************************
   		//Cyclic Data Output
   		//*********************************
   
   		Master_OutputTag.Output_Data136 := DeviceData.OutputData[0];
   		Master_OutputTag.Output_Data137 := DeviceData.OutputData[1];
   		Master_OutputTag.Output_Data138 := DeviceData.OutputData[2];
   		Master_OutputTag.Output_Data139 := DeviceData.OutputData[3];
   		Master_OutputTag.Output_Data140 := DeviceData.OutputData[4];
   		Master_OutputTag.Output_Data141 := DeviceData.OutputData[5];
   		Master_OutputTag.Output_Data142 := DeviceData.OutputData[6];
   		Master_OutputTag.Output_Data143 := DeviceData.OutputData[7];
   		Master_OutputTag.Output_Data144 := DeviceData.OutputData[8];
   		Master_OutputTag.Output_Data145 := DeviceData.OutputData[9];
   		Master_OutputTag.Output_Data146 := DeviceData.OutputData[10];
   		Master_OutputTag.Output_Data147 := DeviceData.OutputData[11];
   		Master_OutputTag.Output_Data148 := DeviceData.OutputData[12];
   		Master_OutputTag.Output_Data149 := DeviceData.OutputData[13];
   		Master_OutputTag.Output_Data150 := DeviceData.OutputData[14];
   		Master_OutputTag.Output_Data151 := DeviceData.OutputData[15];
   
   	else
   
   
   
   end_case;
   
   if CommAOIBusy = 0 then
   
   	DeviceData.OldState := 0;
   	DeviceData.CommSuccess := 0;
   	DeviceData.CommTimeOut := 0;
   	DeviceData.ReplayIndex := 0;
   	DataSendExecuted := 0;
   	DataSendExecuted :=0;
   	ExecuteCounter := 0;
   
   end_if;
   
   if Send_Request > 0 and CommAOIBusy = 0 then
   
   	CommAOIBusy := 1;
   
   	for cChannel := 0 to 8 do
   
   		if Send_Request.[cChannel] then
   
   			ActiveComPort := cChannel;
   
   			exit;
   
   		end_if;
   
   	end_for;
   
   end_if;
   
   if CommAOIBusy = 1
   	and DeviceData.DevicePort = ActiveComPort
   	and DeviceData.StateDone
   	and DeviceData.State > 0
   	and not DataSendExecuted then
   
   	ExecuteCounter := ExecuteCounter +1;
   
   	Master_OutputTag.Output_Data6 .7 := 0;
   	DeviceData.CommSuccess := 0;
   	DeviceData.CommTimeOut := 0;
   
   	Master_OutputTag.Output_Data3 := DataToSend[2];		//iDevice_Port;
   	Master_OutputTag.Output_Data4 := DataToSend[3];		//CMD_Index;
   	Master_OutputTag.Output_Data5 := DataToSend[4];		//CMD_Subindex;
   	Master_OutputTag.Output_Data6.0 := DataToSend[5].0;	//CMD_Rd;
   	Master_OutputTag.Output_Data6.1 := DataToSend[5].1;	//CMD_Wr;
   	Master_OutputTag.Output_Data6.8 := DataToSend[5].8;	//CMD_ByteLength.0;  // Bits für die Länge
   	Master_OutputTag.Output_Data6.9 := DataToSend[5].9;	//CMD_ByteLength.1;
   	Master_OutputTag.Output_Data6.10 := DataToSend[5].10;	//CMD_ByteLength.2;
   	Master_OutputTag.Output_Data6.11 := DataToSend[5].11;	//CMD_ByteLength.3;
   	Master_OutputTag.Output_Data6.12 := DataToSend[5].12;	//CMD_ByteLength.4;
   	Master_OutputTag.Output_Data6.13 := DataToSend[5].13;	//CMD_ByteLength.5;
   	Master_OutputTag.Output_Data6.14 := DataToSend[5].14;	//CMD_ByteLength.6;
   	Master_OutputTag.Output_Data6.15 := DataToSend[5].15;	//CMD_ByteLength.7;
   	Master_OutputTag.Output_Data7 := DataToSend[6];
   	Master_OutputTag.Output_Data8 := DataToSend[7];
   	Master_OutputTag.Output_Data9 := DataToSend[8];
   	Master_OutputTag.Output_Data10 := DataToSend[9];
   
   	Master_OutputTag.Output_Data6.7 := DataToSend[5].7;	//Trigger
   
   	DataSendExecuted :=1;
   
   	CommError.0	:= Master_InputTag.Input_Data6.8;
   	CommError.1	:= Master_InputTag.Input_Data6.9;
   	CommError.2	:= Master_InputTag.Input_Data6.10;
   	CommError.3	:= Master_InputTag.Input_Data6.11;
   	CommError.4	:= Master_InputTag.Input_Data6.12;
   	CommError.5	:= Master_InputTag.Input_Data6.13;
   	CommError.6	:= Master_InputTag.Input_Data6.14;
   	CommError.7	:= Master_InputTag.Input_Data6.15;
   
   	DeviceData.NewState := 0;
   
   	if CommError >0 and DataToSend[3] = Master_InputTag.Input_Data4 then
   
   		DeviceData.AOI_Diagnostic.[DeviceData.State+7] := 1;
   
   	end_if;
   
   end_if;
   
   //*********************************************************************
   // Read or write to check if read or write to check for skipped steps
   //*********************************************************************
   
   RW_Input.0 := Master_InputTag.Input_Data6.0;
   RW_Input.1 := Master_InputTag.Input_Data6.1;
   
   RW_Step.0 := DataToSend[5].0;
   RW_Step.1 := DataToSend[5].1;
   
   //*********************************
   //Acyclic Data
   //*********************************
   
   if Master_InputTag.Input_Data6.7
   
   	and DeviceData.DevicePort = ActiveComPort
   	and Master_InputTag.Input_Data4 = Master_OutputTag.Output_Data4
   	and DeviceData.State > DeviceData.OldState
   	and RW_Input = RW_Step
   	and DataSendExecuted
   	and DeviceData.State > 0  then
   
       DataSendExecuted :=0;
   	DataSize.0 :=	Master_InputTag.Input_Data7.0;
   	DataSize.1 :=	Master_InputTag.Input_Data7.1;
   	DataSize.2 :=	Master_InputTag.Input_Data7.2;
   	DataSize.3 :=	Master_InputTag.Input_Data7.3;
   	DataSize.4 :=	Master_InputTag.Input_Data7.4;
   	DataSize.5 :=	Master_InputTag.Input_Data7.5;
   	DataSize.6 :=	Master_InputTag.Input_Data7.6;
   	DataSize.7 :=	Master_InputTag.Input_Data7.7;
   
   	case DataSize of
   
   		0:
   		DeviceData.AcyclicData[0] := 0;
   
   		DeviceData.CommSuccess := 1;
   		DeviceData.StateDone := 0;
   		Master_OutputTag.Output_Data6.7 := 0;
   
   		DeviceData.ReplayIndex := Master_InputTag.Input_Data4;
   
   
   		1:
   		DeviceData.AcyclicData[0].0 := Master_InputTag.Input_Data7.8;
   		DeviceData.AcyclicData[0].1 := Master_InputTag.Input_Data7.9;
   		DeviceData.AcyclicData[0].2 := Master_InputTag.Input_Data7.10;
   		DeviceData.AcyclicData[0].3 := Master_InputTag.Input_Data7.11;
   		DeviceData.AcyclicData[0].4 := Master_InputTag.Input_Data7.12;
   		DeviceData.AcyclicData[0].5 := Master_InputTag.Input_Data7.13;
   		DeviceData.AcyclicData[0].6 := Master_InputTag.Input_Data7.14;
   		DeviceData.AcyclicData[0].7 := Master_InputTag.Input_Data7.15;
   
   		DeviceData.CommSuccess := 1;
   		DeviceData.StateDone := 0;
   		Master_OutputTag.Output_Data6.7 := 0;
   
   		DeviceData.ReplayIndex := Master_InputTag.Input_Data4;
   
   		2:
   		DeviceData.AcyclicData[0].0 := Master_InputTag.Input_Data8.0;
   		DeviceData.AcyclicData[0].1 := Master_InputTag.Input_Data8.1;
   		DeviceData.AcyclicData[0].2 := Master_InputTag.Input_Data8.2;
   		DeviceData.AcyclicData[0].3 := Master_InputTag.Input_Data8.3;
   		DeviceData.AcyclicData[0].4 := Master_InputTag.Input_Data8.4;
   		DeviceData.AcyclicData[0].5 := Master_InputTag.Input_Data8.5;
   		DeviceData.AcyclicData[0].6 := Master_InputTag.Input_Data8.6;
   		DeviceData.AcyclicData[0].7 := Master_InputTag.Input_Data8.7;
   		DeviceData.AcyclicData[0].8 := Master_InputTag.Input_Data7.8;
   		DeviceData.AcyclicData[0].9 := Master_InputTag.Input_Data7.9;
   		DeviceData.AcyclicData[0].10 := Master_InputTag.Input_Data7.10;
   		DeviceData.AcyclicData[0].11 := Master_InputTag.Input_Data7.11;
   		DeviceData.AcyclicData[0].12 := Master_InputTag.Input_Data7.12;
   		DeviceData.AcyclicData[0].13 := Master_InputTag.Input_Data7.13;
   		DeviceData.AcyclicData[0].14 := Master_InputTag.Input_Data7.14;
   		DeviceData.AcyclicData[0].15 := Master_InputTag.Input_Data7.15;
   
   		DeviceData.CommSuccess := 1;
   		DeviceData.StateDone := 0;
   		Master_OutputTag.Output_Data6.7 := 0;
   
   		DeviceData.ReplayIndex := Master_InputTag.Input_Data4;
   
   		4:
   
   		DeviceData.AcyclicData[0].0 := Master_InputTag.Input_Data9.0;
   		DeviceData.AcyclicData[0].1 := Master_InputTag.Input_Data9.1;
   		DeviceData.AcyclicData[0].2 := Master_InputTag.Input_Data9.2;
   		DeviceData.AcyclicData[0].3 := Master_InputTag.Input_Data9.3;
   		DeviceData.AcyclicData[0].4 := Master_InputTag.Input_Data9.4;
   		DeviceData.AcyclicData[0].5 := Master_InputTag.Input_Data9.5;
   		DeviceData.AcyclicData[0].6 := Master_InputTag.Input_Data9.6;
   		DeviceData.AcyclicData[0].7 := Master_InputTag.Input_Data9.7;
   		DeviceData.AcyclicData[0].8 :=  Master_InputTag.Input_Data8.8;
   		DeviceData.AcyclicData[0].9 :=  Master_InputTag.Input_Data8.9;
   		DeviceData.AcyclicData[0].10 := Master_InputTag.Input_Data8.10;
   		DeviceData.AcyclicData[0].11 := Master_InputTag.Input_Data8.11;
   		DeviceData.AcyclicData[0].12 := Master_InputTag.Input_Data8.12;
   		DeviceData.AcyclicData[0].13 := Master_InputTag.Input_Data8.13;
   		DeviceData.AcyclicData[0].14 := Master_InputTag.Input_Data8.14;
   		DeviceData.AcyclicData[0].15 := Master_InputTag.Input_Data8.15;
   	 	DeviceData.AcyclicData[0].16 := Master_InputTag.Input_Data8.0;
   		DeviceData.AcyclicData[0].17 := Master_InputTag.Input_Data8.1;
   		DeviceData.AcyclicData[0].18 := Master_InputTag.Input_Data8.2;
   		DeviceData.AcyclicData[0].19 := Master_InputTag.Input_Data8.3;
   		DeviceData.AcyclicData[0].20 := Master_InputTag.Input_Data8.4;
   		DeviceData.AcyclicData[0].21 := Master_InputTag.Input_Data8.5;
   		DeviceData.AcyclicData[0].22 := Master_InputTag.Input_Data8.6;
   		DeviceData.AcyclicData[0].23 := Master_InputTag.Input_Data8.7;
   		DeviceData.AcyclicData[0].24 := Master_InputTag.Input_Data7.8;
   		DeviceData.AcyclicData[0].25 := Master_InputTag.Input_Data7.9;
   		DeviceData.AcyclicData[0].26 := Master_InputTag.Input_Data7.10;
   		DeviceData.AcyclicData[0].27 := Master_InputTag.Input_Data7.11;
   		DeviceData.AcyclicData[0].28 := Master_InputTag.Input_Data7.12;
   		DeviceData.AcyclicData[0].29 := Master_InputTag.Input_Data7.13;
   		DeviceData.AcyclicData[0].30 := Master_InputTag.Input_Data7.14;
   		DeviceData.AcyclicData[0].31 := Master_InputTag.Input_Data7.15;
   
   		DeviceData.CommSuccess := 1;
   		DeviceData.StateDone := 0;
   		Master_OutputTag.Output_Data6.7 := 0;
   
   		DeviceData.ReplayIndex := Master_InputTag.Input_Data4;
   
   		6:
   
   		DeviceData.AcyclicData[0].0 := Master_InputTag.Input_Data9.0;
   		DeviceData.AcyclicData[0].1 := Master_InputTag.Input_Data9.1;
   		DeviceData.AcyclicData[0].2 := Master_InputTag.Input_Data9.2;
   		DeviceData.AcyclicData[0].3 := Master_InputTag.Input_Data9.3;
   		DeviceData.AcyclicData[0].4 := Master_InputTag.Input_Data9.4;
   		DeviceData.AcyclicData[0].5 := Master_InputTag.Input_Data9.5;
   		DeviceData.AcyclicData[0].6 := Master_InputTag.Input_Data9.6;
   		DeviceData.AcyclicData[0].7 := Master_InputTag.Input_Data9.7;
   		DeviceData.AcyclicData[0].8 :=  Master_InputTag.Input_Data8.8;
   		DeviceData.AcyclicData[0].9 :=  Master_InputTag.Input_Data8.9;
   		DeviceData.AcyclicData[0].10 := Master_InputTag.Input_Data8.10;
   		DeviceData.AcyclicData[0].11 := Master_InputTag.Input_Data8.11;
   		DeviceData.AcyclicData[0].12 := Master_InputTag.Input_Data8.12;
   		DeviceData.AcyclicData[0].13 := Master_InputTag.Input_Data8.13;
   		DeviceData.AcyclicData[0].14 := Master_InputTag.Input_Data8.14;
   		DeviceData.AcyclicData[0].15 := Master_InputTag.Input_Data8.15;
   	 	DeviceData.AcyclicData[0].16 := Master_InputTag.Input_Data8.0;
   		DeviceData.AcyclicData[0].17 := Master_InputTag.Input_Data8.1;
   		DeviceData.AcyclicData[0].18 := Master_InputTag.Input_Data8.2;
   		DeviceData.AcyclicData[0].19 := Master_InputTag.Input_Data8.3;
   		DeviceData.AcyclicData[0].20 := Master_InputTag.Input_Data8.4;
   		DeviceData.AcyclicData[0].21 := Master_InputTag.Input_Data8.5;
   		DeviceData.AcyclicData[0].22 := Master_InputTag.Input_Data8.6;
   		DeviceData.AcyclicData[0].23 := Master_InputTag.Input_Data8.7;
   		DeviceData.AcyclicData[0].24 := Master_InputTag.Input_Data7.8;
   		DeviceData.AcyclicData[0].25 := Master_InputTag.Input_Data7.9;
   		DeviceData.AcyclicData[0].26 := Master_InputTag.Input_Data7.10;
   		DeviceData.AcyclicData[0].27 := Master_InputTag.Input_Data7.11;
   		DeviceData.AcyclicData[0].28 := Master_InputTag.Input_Data7.12;
   		DeviceData.AcyclicData[0].29 := Master_InputTag.Input_Data7.13;
   		DeviceData.AcyclicData[0].30 := Master_InputTag.Input_Data7.14;
   		DeviceData.AcyclicData[0].31 := Master_InputTag.Input_Data7.15;
   
   		DeviceData.AcyclicData[1].0 := Master_InputTag.Input_Data10.0;
   		DeviceData.AcyclicData[1].1 := Master_InputTag.Input_Data10.1;
   		DeviceData.AcyclicData[1].2 := Master_InputTag.Input_Data10.2;
   		DeviceData.AcyclicData[1].3 := Master_InputTag.Input_Data10.3;
   		DeviceData.AcyclicData[1].4 := Master_InputTag.Input_Data10.4;
   		DeviceData.AcyclicData[1].5 := Master_InputTag.Input_Data10.5;
   		DeviceData.AcyclicData[1].6 := Master_InputTag.Input_Data10.6;
   		DeviceData.AcyclicData[1].7 := Master_InputTag.Input_Data10.7;
   		DeviceData.AcyclicData[1].8 :=  Master_InputTag.Input_Data9.8;
   		DeviceData.AcyclicData[1].9 :=  Master_InputTag.Input_Data9.9;
   		DeviceData.AcyclicData[1].10 := Master_InputTag.Input_Data9.10;
   		DeviceData.AcyclicData[1].11 := Master_InputTag.Input_Data9.11;
   		DeviceData.AcyclicData[1].12 := Master_InputTag.Input_Data9.12;
   		DeviceData.AcyclicData[1].13 := Master_InputTag.Input_Data9.13;
   		DeviceData.AcyclicData[1].14 := Master_InputTag.Input_Data9.14;
   		DeviceData.AcyclicData[1].15 := Master_InputTag.Input_Data9.15;
   
   		DeviceData.CommSuccess := 1;
   		DeviceData.StateDone := 0;
   		Master_OutputTag.Output_Data6.7 := 0;
   
   		DeviceData.ReplayIndex := Master_InputTag.Input_Data4;
   
   		8:
   
   		DeviceData.AcyclicData[0].0 := Master_InputTag.Input_Data9.0;
   		DeviceData.AcyclicData[0].1 := Master_InputTag.Input_Data9.1;
   		DeviceData.AcyclicData[0].2 := Master_InputTag.Input_Data9.2;
   		DeviceData.AcyclicData[0].3 := Master_InputTag.Input_Data9.3;
   		DeviceData.AcyclicData[0].4 := Master_InputTag.Input_Data9.4;
   		DeviceData.AcyclicData[0].5 := Master_InputTag.Input_Data9.5;
   		DeviceData.AcyclicData[0].6 := Master_InputTag.Input_Data9.6;
   		DeviceData.AcyclicData[0].7 := Master_InputTag.Input_Data9.7;
   		DeviceData.AcyclicData[0].8 :=  Master_InputTag.Input_Data8.8;
   		DeviceData.AcyclicData[0].9 :=  Master_InputTag.Input_Data8.9;
   		DeviceData.AcyclicData[0].10 := Master_InputTag.Input_Data8.10;
   		DeviceData.AcyclicData[0].11 := Master_InputTag.Input_Data8.11;
   		DeviceData.AcyclicData[0].12 := Master_InputTag.Input_Data8.12;
   		DeviceData.AcyclicData[0].13 := Master_InputTag.Input_Data8.13;
   		DeviceData.AcyclicData[0].14 := Master_InputTag.Input_Data8.14;
   		DeviceData.AcyclicData[0].15 := Master_InputTag.Input_Data8.15;
   	 	DeviceData.AcyclicData[0].16 := Master_InputTag.Input_Data8.0;
   		DeviceData.AcyclicData[0].17 := Master_InputTag.Input_Data8.1;
   		DeviceData.AcyclicData[0].18 := Master_InputTag.Input_Data8.2;
   		DeviceData.AcyclicData[0].19 := Master_InputTag.Input_Data8.3;
   		DeviceData.AcyclicData[0].20 := Master_InputTag.Input_Data8.4;
   		DeviceData.AcyclicData[0].21 := Master_InputTag.Input_Data8.5;
   		DeviceData.AcyclicData[0].22 := Master_InputTag.Input_Data8.6;
   		DeviceData.AcyclicData[0].23 := Master_InputTag.Input_Data8.7;
   		DeviceData.AcyclicData[0].24 := Master_InputTag.Input_Data7.8;
   		DeviceData.AcyclicData[0].25 := Master_InputTag.Input_Data7.9;
   		DeviceData.AcyclicData[0].26 := Master_InputTag.Input_Data7.10;
   		DeviceData.AcyclicData[0].27 := Master_InputTag.Input_Data7.11;
   		DeviceData.AcyclicData[0].28 := Master_InputTag.Input_Data7.12;
   		DeviceData.AcyclicData[0].29 := Master_InputTag.Input_Data7.13;
   		DeviceData.AcyclicData[0].30 := Master_InputTag.Input_Data7.14;
   		DeviceData.AcyclicData[0].31 := Master_InputTag.Input_Data7.15;
   
   		DeviceData.AcyclicData[1].0 := Master_InputTag.Input_Data11.0;
   		DeviceData.AcyclicData[1].1 := Master_InputTag.Input_Data11.1;
   		DeviceData.AcyclicData[1].2 := Master_InputTag.Input_Data11.2;
   		DeviceData.AcyclicData[1].3 := Master_InputTag.Input_Data11.3;
   		DeviceData.AcyclicData[1].4 := Master_InputTag.Input_Data11.4;
   		DeviceData.AcyclicData[1].5 := Master_InputTag.Input_Data11.5;
   		DeviceData.AcyclicData[1].6 := Master_InputTag.Input_Data11.6;
   		DeviceData.AcyclicData[1].7 := Master_InputTag.Input_Data11.7;
   		DeviceData.AcyclicData[1].8 :=  Master_InputTag.Input_Data10.8;
   		DeviceData.AcyclicData[1].9 :=  Master_InputTag.Input_Data10.9;
   		DeviceData.AcyclicData[1].10 := Master_InputTag.Input_Data10.10;
   		DeviceData.AcyclicData[1].11 := Master_InputTag.Input_Data10.11;
   		DeviceData.AcyclicData[1].12 := Master_InputTag.Input_Data10.12;
   		DeviceData.AcyclicData[1].13 := Master_InputTag.Input_Data10.13;
   		DeviceData.AcyclicData[1].14 := Master_InputTag.Input_Data10.14;
   		DeviceData.AcyclicData[1].15 := Master_InputTag.Input_Data10.15;
   	 	DeviceData.AcyclicData[1].16 := Master_InputTag.Input_Data10.0;
   		DeviceData.AcyclicData[1].17 := Master_InputTag.Input_Data10.1;
   		DeviceData.AcyclicData[1].18 := Master_InputTag.Input_Data10.2;
   		DeviceData.AcyclicData[1].19 := Master_InputTag.Input_Data10.3;
   		DeviceData.AcyclicData[1].20 := Master_InputTag.Input_Data10.4;
   		DeviceData.AcyclicData[1].21 := Master_InputTag.Input_Data10.5;
   		DeviceData.AcyclicData[1].22 := Master_InputTag.Input_Data10.6;
   		DeviceData.AcyclicData[1].23 := Master_InputTag.Input_Data10.7;
   		DeviceData.AcyclicData[1].24 := Master_InputTag.Input_Data9.8;
   		DeviceData.AcyclicData[1].25 := Master_InputTag.Input_Data9.9;
   		DeviceData.AcyclicData[1].26 := Master_InputTag.Input_Data9.10;
   		DeviceData.AcyclicData[1].27 := Master_InputTag.Input_Data9.11;
   		DeviceData.AcyclicData[1].28 := Master_InputTag.Input_Data9.12;
   		DeviceData.AcyclicData[1].29 := Master_InputTag.Input_Data9.13;
   		DeviceData.AcyclicData[1].30 := Master_InputTag.Input_Data9.14;
   		DeviceData.AcyclicData[1].31 := Master_InputTag.Input_Data9.15;
   
   		DeviceData.CommSuccess := 1;
   		DeviceData.StateDone := 0;
   		Master_OutputTag.Output_Data6.7 := 0;
   
   		DeviceData.ReplayIndex := Master_InputTag.Input_Data4;
   
   	end_case;
   
   end_if;
   
END_ROUTINE
END_ADD_ON_INSTRUCTION
